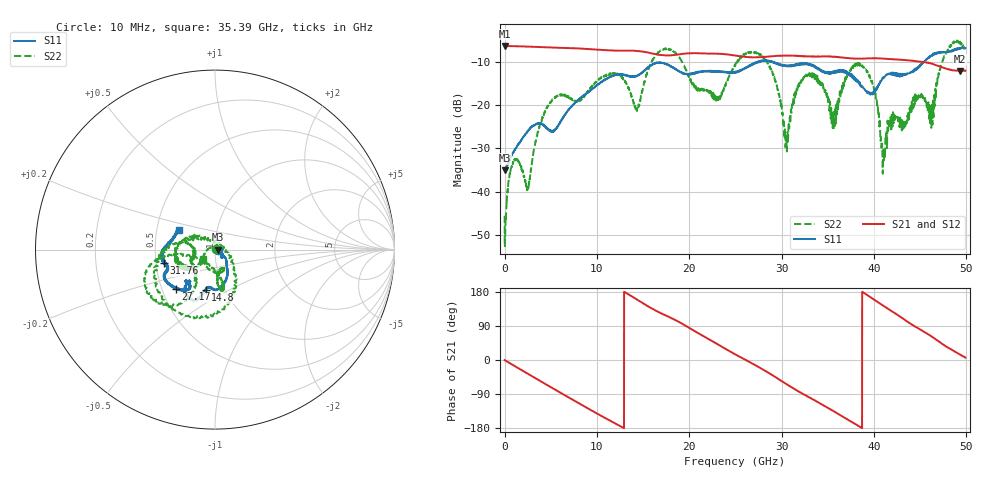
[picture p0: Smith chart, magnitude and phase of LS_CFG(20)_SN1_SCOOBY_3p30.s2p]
!Keysight Technologies,N5245B,MY58422026,A.13.80.08
!Date: Thursday, March 19, 2020 23:32:59
!Correction: S11(Full 2 Port(1,2))
!S21(Full 2 Port(1,2))
!S12(Full 2 Port(1,2))
!S22(Full 2 Port(1,2))
!S2P File: Measurements: S11, S21, S12, S22:
# Hz S DB R 50.0
!freq dBS11 angS11 dBS21 angS21 dBS12 angS12 dBS22 angS22
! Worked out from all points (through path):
!   4991 points, 10 MHz to 49.91 GHz, reference 50 ohm
!   highest |S21| = -6.39 dB at 10 MHz (marker M1); lowest = -12.1 dB at 49.35 GHz (marker M2)
!   group delay of S21, straight-line fit = 39.3 ps
!   lowest |S11| = -35.1 dB at 50 MHz (marker M3), VSWR 1.04, Z = 51.8 + j0.00317 ohm
!   |S11| at or under -10 dB: start of sweep to 27.5 GHz; 28.8856 GHz to 28.95115 GHz (65.56 MHz wide, 0.227 % of centre); 29 GHz to 45.4 GHz (16.4 GHz wide, 44.1 % of centre)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
!   |S22| runs from -52.6 to -5.1 dB; largest |S21 - S12| = 0.0045
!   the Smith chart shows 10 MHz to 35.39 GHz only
!   S11 on the Smith chart (normalised r, x): 10 MHz: 1.04, -0.01; 14.8 GHz: 0.82, -0.39; 27.17 GHz: 0.59, -0.29; 31.76 GHz: 0.55, -0.09; 35.39 GHz: 0.65, +0.15
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1e7  -35.00 -10.7  -6.39 -0.3  -6.37 -0.3  -45.55 14.1
5e7  -35.10 0.1  -6.39 -0.8  -6.39 -0.8  -51.92 -55.0
8.6e8  -31.14 -15.8  -6.45 -12.5  -6.44 -12.5  -33.40 -73.9
2.53e9  -26.11 -30.8  -6.55 -36.4  -6.55 -36.4  -39.13 75.3
4.78e9  -25.58 -50.4  -6.72 -68.3  -6.72 -68.3  -20.03 -123.6
8.33e9  -18.33 -56.8  -7.01 -118.0  -7.00 -118.0  -18.63 -76.6
1.48e10  -12.69 -103.1  -7.63 152.5  -7.62 152.5  -18.03 -159.8
1.665e10  -10.27 -114.5  -8.41 126.9  -8.40 126.9  -7.93 -161.8
2.299e10  -12.38 -129.4  -8.17 42.9  -8.18 43.0  -19.16 -168.3
2.496e10  -12.52 -128.9  -8.58 15.2  -8.57 15.3  -10.95 -176.9
2.717e10  -10.18 -134.6  -9.01 -13.8  -9.00 -13.7  -7.92 -113.2
3.05e10  -11.01 -159.0  -8.62 -63.2  -8.62 -63.0  -27.70 45.3
3.176e10  -10.68 -165.4  -8.73 -81.8  -8.73 -81.5  -15.53 157.5
3.328e10  -10.76 179.0  -8.82 -102.6  -8.82 -102.3  -12.85 -161.9
3.539e10  -12.78 151.7  -8.85 -131.7  -8.80 -131.4  -21.51 -141.1
3.841e10  -15.02 114.2  -9.35 -175.3  -9.30 -175.7  -10.34 -155.3
3.997e10  -17.39 78.6  -9.23 160.2  -9.21 159.9  -15.70 -100.7
4.096e10  -13.77 55.5  -9.30 144.1  -9.33 143.8  -35.86 20.4
4.16e10  -12.74 48.0  -9.41 134.1  -9.43 133.9  -23.71 123.9
4.625e10  -8.58 -18.9  -10.49 61.9  -10.52 61.8  -21.92 143.7
4.935e10  -6.89 -45.3  -12.14 14.0  -12.15 14.0  -5.46 -29.3
4.991e10  -6.93 -42.6  -12.08 6.4  -12.11 6.3  -7.51 -15.3
